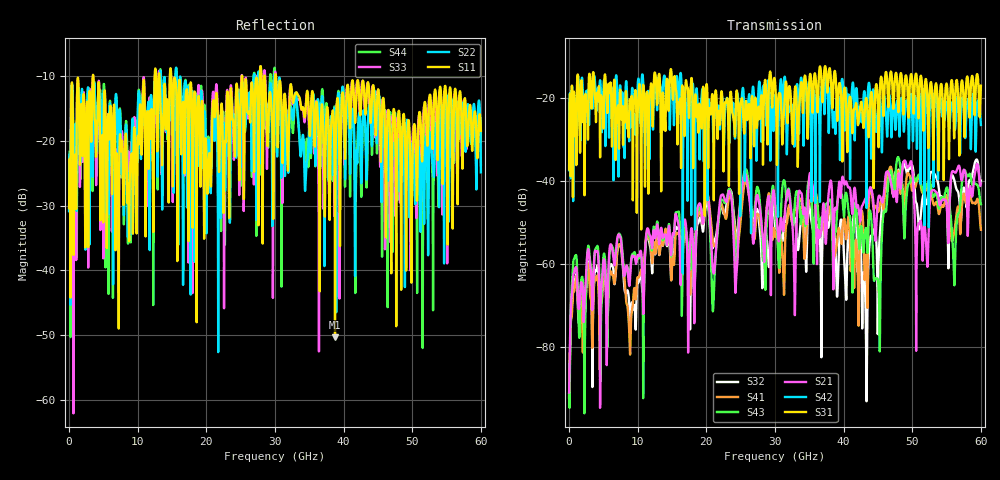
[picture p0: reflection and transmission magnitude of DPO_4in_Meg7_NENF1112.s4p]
! Tyco Electronics Strada Whisper System
! NEXT_F1112_G1112
!! SYSTEM DESCRIPTION: Daughtercard-Footprint-Connector-Footprint-Daughtercard
!! PCB DESCRIPTION: DC: 140mil, Megtron7N, upper layer route, 15mil stub, 6-6-6mil 4" traces
!! CONNECTOR DESCRIPTION: Next-Gen STRADA Whisper Direct-Plug Orthogonal Connector
!! MODEL DESCRIPTION: Tyco Electronics System 4-port S-parameter
!! MODEL STATUS: Developmental
!! MODEL GEOMETRY: Channel Model
!! MODEL FREQUENCY RANGE: DC to 60 GHz in 10 MHz frequency steps
!! MODEL EDGE RATE LIMITATION: 8.3 ps (Using conservative 0.5/Fmax rule of thumb)
!! TIME-DOMAIN TRANSFORM CAUTIONS:
!! 1.) Do not simulate transient edge rates faster than the number listed above.  Edge rates faster than this number
!!  contain significant spectral content at frequencies above the model's highest frequency.
!! 2.) Even when simulating edge rates that are slower than the number listed above, be aware that the best time
!!  resolution possible with a direct iFFT is (1 / 2Fmax).  As a result, time resolution is typically not adequate
!!  for most time-domain simulations unless tricks such as windowing are used to minimize leakage and aliasing.
!! 3.) Because the model has a uniform frequency step, a direct iFFT will result in an impulse that that has a time
!!  length given by either (1 / Fstep) or (1 / 2Fstep), depending on the transform being used.  Care has been taken
!!  in selecting the frequency step to ensure a settled impulse response for the model.  Therefore, convolution with
!!  the model's impulse response should present no issues.  However, if directly concatenating s-parameter models
!!  in the frequency domain a user must either interpolate necessary interim frequencies or complete impulse response
!!  zero-padding.  Impulse response zero-padding is more difficult, but more accurate.
!! PORT DEFINITIONS:
!! Port  1  ----->  RX Side	F11  G11  RX Side  <-----  Port  3
!! Port  2  ----->  RX Side	F12  G12  RX Side  <-----  Port  4
! Touchstone data
! Created: 10-Dec-2018 by IdEM R2012 (8.0.5)
# Hz S MA R 50
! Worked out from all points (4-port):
!   6000 points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, 10 MHz to 60 GHz, reference 50 ohm
!   strongest paths, dB at 10 MHz, 15.01 GHz, 30.01 GHz, 45.01 GHz, 60 GHz:
!     S31: -37.1, -16.4, -16.0, -23.8, -17.0
!     S42: -37.3, -16.6, -19.7, -22.7, -26.4
!     S21: -90.9, -54.2, -45.3, -44.5, -40.5
!     S43: -91.3, -55.0, -47.5, -63.9, -45.5
!     S41: -91.7, -59.8, -53.4, -47.3, -51.7
!     S32: -92.2, -59.0, -51.0, -69.7, -39.8
!   lowest |S11| = -50.3 dB at 38.75 GHz (marker M1), VSWR 1.01, Z = 49.7 + j0.0608 ohm
!   |S11| at or under -10 dB: 3.53 GHz to 12.48 GHz (8.954 GHz wide, 112 % of centre); 14.89 GHz to 25.19 GHz (10.3 GHz wide, 51.4 % of centre); 30.13 GHz to end of sweep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
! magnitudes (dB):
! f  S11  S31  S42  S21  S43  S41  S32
! 10 MHz  -30.4  -37.1  -37.3  -90.9  -91.3  -91.7  -92.2
! 20 GHz  -21.9  -17.1  -17.7  -43.5  -43.9  -43.9  -45.5
! 21.01 GHz  -13.8  -24.7  -29.9  -61.9  -70.5  -55.2  -55.6
! 25.72 GHz  -10.7  -21.2  -26.1  -38.4  -37.2  -40.2  -38.5
! 28.41 GHz  -10.6  -18.9  -17.1  -59.3  -58.5  -55.9  -54.9
! 38.75 GHz  -50.3  -13.5  -26.0  -46.5  -51.8  -57.4  -54.1
! 60 GHz  -18.5  -17.0  -26.4  -40.5  -45.5  -51.7  -39.8
